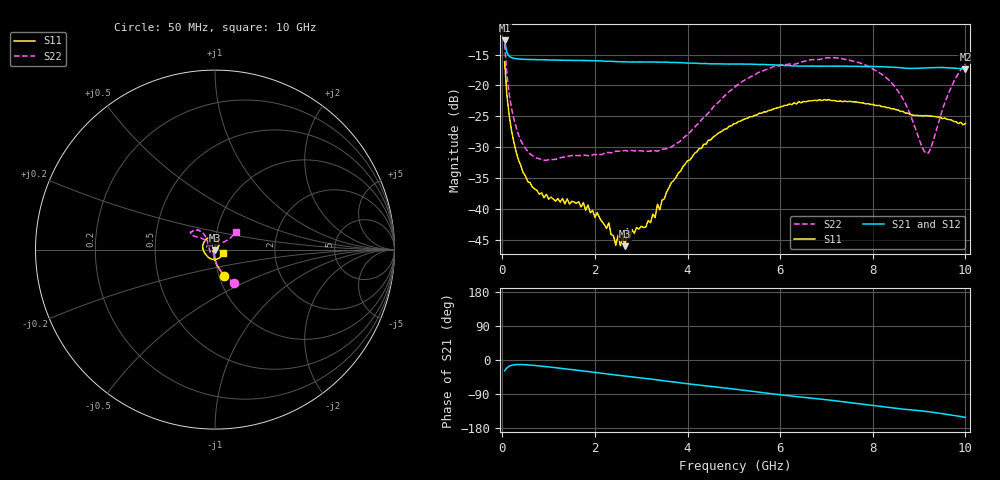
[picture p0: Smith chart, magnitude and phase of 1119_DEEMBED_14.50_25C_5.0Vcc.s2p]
!Hittite Microwave Corp.
!Digital Attenuator/PhaseShifter Rev 1.4.0
!Filename: C:\DATA\DATA\1119_DEEMBED_14.50_25C_5.0Vcc.s2p
!VNA ID: Agilent Technologies,N5224A,MY51441122,A.10.45.03
!Device type:
!2 Port Calibration.
!Temp(C): 25
!Lot Number:
!Serial Number:
!Operator:
!Misc:
!Attenuator:  14.500
# GHZ S DB R 50.0
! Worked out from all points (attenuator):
!   200 points, 50 MHz to 10 GHz, reference 50 ohm
!   highest |S21| = -12.72 dB at 50 MHz (marker M1); lowest = -17.4 dB at 10 GHz (marker M2)
!   lowest |S11| = -46.1 dB at 2.65 GHz (marker M3), VSWR 1.01, Z = 50.1 - j0.493 ohm
!   |S11| at or under -10 dB: start of sweep to end of sweep
!   |S22| runs from -32.1 to -13.3 dB; largest |S21 - S12| = 0.0004
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0.05  -16.18 -71.4  -12.72 -28.6  -12.72 -28.6  -13.31 -60.6
0.1  -21.63 -84.2  -14.70 -20.8  -14.70 -20.8  -18.22 -75.4
0.2  -27.38 -95.5  -15.50 -14.0  -15.50 -13.9  -23.73 -86.8
0.35  -32.10 -105.9  -15.72 -12.0  -15.72 -12.0  -28.01 -93.9
0.55  -35.63 -119.1  -15.80 -12.9  -15.80 -12.9  -30.70 -100.0
0.9  -38.22 -132.2  -15.86 -16.9  -15.86 -16.9  -32.13 -106.3
1.75  -39.01 -137.7  -15.97 -29.0  -15.97 -29.1  -31.33 -115.9
2.3  -42.31 -127.8  -16.09 -37.3  -16.08 -37.4  -30.89 -131.2
2.45  -45.93 -109.4  -16.15 -39.6  -16.15 -39.6  -30.69 -134.5
2.5  -44.30 -102.5  -16.16 -40.3  -16.16 -40.4  -30.68 -135.7
2.65  -46.08 -82.1  -16.20 -42.4  -16.20 -42.4  -30.57 -140.9
2.7  -43.26 -70.5  -16.20 -43.0  -16.20 -43.1  -30.65 -141.8
2.75  -44.80 -68.9  -16.21 -43.7  -16.22 -43.8  -30.55 -144.0
3.4  -40.18 13.0  -16.23 -53.3  -16.24 -53.3  -30.53 -175.9
4  -32.24 41.9  -16.39 -62.5  -16.40 -62.6  -28.05 150.1
5.05  -26.17 71.0  -16.55 -77.3  -16.56 -77.4  -20.10 125.8
6.7  -22.50 121.9  -16.87 -100.8  -16.88 -100.9  -15.83 139.8
7.65  -22.70 156.0  -16.92 -114.5  -16.93 -114.5  -16.19 147.9
8.35  -23.61 -179.0  -17.04 -125.2  -17.04 -125.2  -19.16 142.3
9.2  -24.96 -115.5  -17.16 -136.4  -17.17 -136.4  -30.98 81.8
9.6  -25.49 -73.9  -17.14 -143.5  -17.15 -143.5  -21.96 38.4
10  -26.19 -22.3  -17.39 -151.2  -17.39 -151.2  -16.39 39.6
